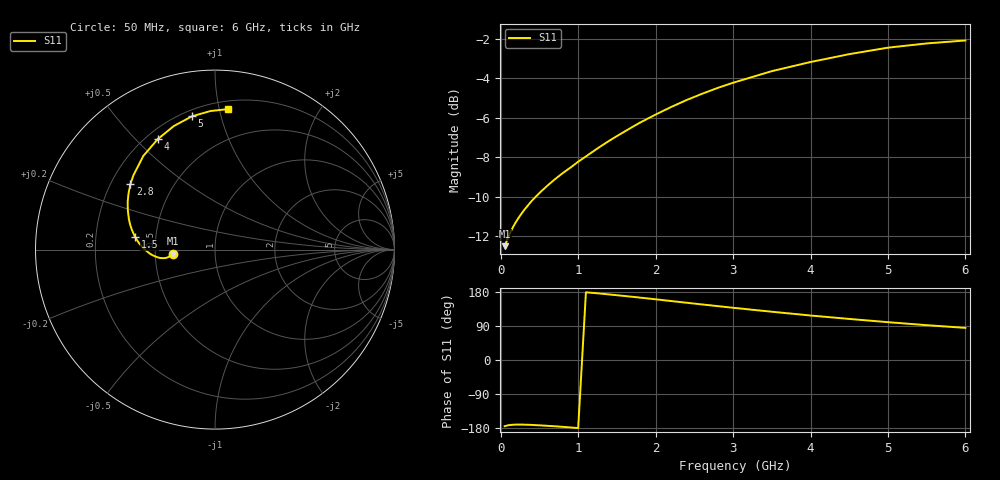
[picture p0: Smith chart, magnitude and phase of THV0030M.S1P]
! SIEMENS Discrete & RF Semiconductors
! BAS70
! Si Schottky Diode in SOT23
! IF = 30 mA
! S-Parameters:  February  1997
# GHz  S  MA  R  50
!  f  S11
! GHz  MAG  ANG
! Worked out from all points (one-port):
!   34 points, 50 MHz to 6 GHz, reference 50 ohm
!   lowest |S11| = -12.5 dB at 50 MHz (marker M1), VSWR 1.62, Z = 30.9 - j1.46 ohm
!   |S11| at or under -10 dB: start of sweep to 451.2 MHz
!   S11 on the Smith chart (normalised r, x): 50 MHz: 0.62, -0.03; 1.5 GHz: 0.38, +0.07; 2.8 GHz: 0.28, +0.32; 4 GHz: 0.25, +0.58; 5 GHz: 0.24, +0.81; 6 GHz: 0.26, +1.06
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0.05  0.2373 -174.6
0.1  0.251 -172.1
0.15  0.2633 -170.9
0.2  0.274 -170.4
0.3  0.2925 -170.6
0.4  0.3089 -171.3
0.5  0.3234 -172.4
0.7  0.3504 -174.9
0.8  0.363 -176.4
1  0.3879 -179.6
1.2  0.4128 176.9
1.3  0.4255 175.0
1.5  0.4504 171.0
1.6  0.4625 168.9
1.7  0.475 166.8
1.8  0.4873 164.6
2  0.5105 160.2
2.2  0.5335 155.6
2.4  0.5556 151.1
2.6  0.5762 146.6
2.8  0.5961 142.2
3  0.6145 137.8
3.5  0.6573 127.4
4  0.6932 117.4
4.5  0.7258 108.4
5  0.7537 99.8
5.5  0.7724 91.9
6  0.786 84.8
